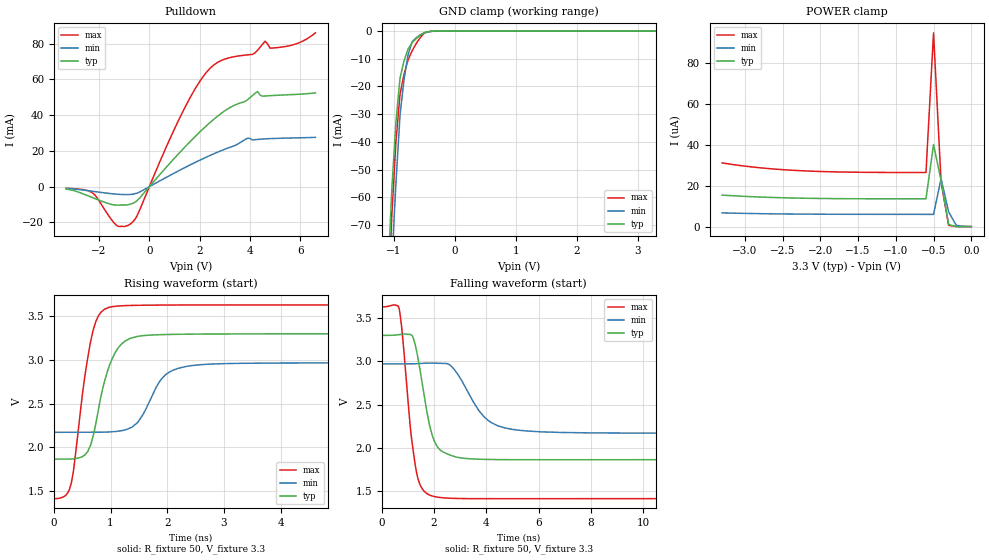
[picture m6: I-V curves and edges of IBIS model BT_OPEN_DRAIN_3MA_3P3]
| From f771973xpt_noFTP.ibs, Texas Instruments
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|   Model Cell BT_OPEN_DRAIN_3MA_3P3
|BT_OPEN_DRAIN_3MA_3P3
[Model]   BT_OPEN_DRAIN_3MA_3P3
Model_type   I/O_open_drain
Polarity   Inverting
Enable   Active-Low
Vinl =  0.8
Vinh =  2
Cref =  15.0000pF
Rref =  100.0000M
Vref =  0V
Vmeas =  1.65
C_comp   3.98845p   2.03906p   4.55356p
[Model Spec]
Vinl   0.8   0.8   0.8
Vinh   2   2   2
[Temperature Range]   25   155   -40
[Voltage Range]   3.3   2.97   3.63
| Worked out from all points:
|   slope of the pulldown table from 0 to 0.495 V, typ, clamps not added: 61.7 ohm
|   GND clamp passes 1 mA (typ) near -0.53 V on its own axis
|   rising waveform, R_fixture 50, V_fixture 3.3: 20-80 % time 326ps typ, 410ps min, 271ps max; typ from 1.87 V to 3.3 V
|   falling waveform, R_fixture 50, V_fixture 3.3: 20-80 % time 525ps typ, 1.02ns min, 426ps max; typ from 3.3 V to 1.86 V
| Nom Voltages:
|   BIASFET=3.3, VDD=1.2, VDDS=3.3, VSS=0
| Min Voltages:
|   BIASFET=2.97, VDD=1.08, VDDS=2.97, VSS=0
| Max Voltages:
|   BIASFET=3.63, VDD=1.32, VDDS=3.63, VSS=0
[POWER_clamp]
|   voltage   I(typ)   I(min)   I(max)
-3.3V     15.41uA    6.707uA    31.17uA
-2.8V     14.47uA    6.332uA    28.78uA
-2.2V     13.87uA    6.102uA    27.25uA
-1.6V     13.64uA    6.016uA    26.64uA
-600mV    13.58uA    5.99uA     26.46uA
-500mV    40.13uA    5.991uA    94.82uA
-400mV    22.54uA    23.52uA    21.76uA
-300mV    969.1nA    7.215uA    616.4nA
-200mV    29.93nA    661.1nA    11.88nA
0V        1.388nA    48.32nA    1.243nA
[Pulldown]
|   voltage   I(typ)   I(min)   I(max)
-3.3V     -1.368mA   -936.2uA   -859.1uA
-2.3V     -5.876mA   -2.477mA   -3.094mA
-1.3V     -10.31mA   -4.18mA    -21.72mA
-800mV    -9.945mA   -4.384mA   -21.31mA
-500mV    -7.961mA   -3.661mA   -16.65mA
1.4V      21.97mA    10.6mA     43.88mA
2.4V      35.71mA    17.39mA    65.97mA
4.3V      53.2mA     26.41mA    76.22mA
4.6V      50.69mA    26.72mA    81.32mA
4.8V      50.87mA    26.86mA    77.39mA
5.4V      51.3mA     27.13mA    78.32mA
6.6V      52.45mA    27.57mA    85.99mA
[GND_clamp]
|   voltage   I(typ)   I(min)   I(max)
-3.3V     -1.746A    -1.481A    -2.454A
-1.1V     -88.72mA   -114.8mA   -101.4mA
-1.033V   -56.66mA   -82.94mA   -65.99mA
-966.7mV  -32.75mA   -54.79mA   -39.79mA
-900mV    -16.98mA   -30.37mA   -22.81mA
-833.3mV  -10.67mA   -17.32mA   -15.58mA
-766.7mV  -6.402mA   -8.477mA   -10.34mA
-700mV    -4.171mA   -3.846mA   -7.085mA
-566.7mV  -1.511mA   -1.331mA   -2.329mA
-500mV    -537.7uA   -639.3uA   -683uA
-300mV    -1.439uA   -12.56uA   -707.1nA
3.3V      1.388nA    14.18uA    1.029nA
[Ramp]
| variable   typ   min   max
dV/dt_f 0.87243134/0.53137713n 0.48603643/1.0377786n   1.344851/0.42962575n
dV/dt_r 0.81373668/0.78906954n 0.45222846/1.5290324n  1.2226949/0.57631885n
R_load = 50
[Rising Waveform]
R_fixture = 50
V_fixture = 3.3
V_fixture_min = 2.97
V_fixture_max = 3.63
|   time   V(typ)   V(min)   V(max)
0s        1.866V     2.173V     1.413V
210.5ps   1.866V     2.173V     1.452V
308.7ps   1.868V     2.173V     1.593V
599.8ps   1.954V     2.173V     3.032V
785.8ps   2.43V      2.173V     3.504V
1.038ns   3.027V     2.179V     3.611V
1.48ns    3.27V      2.287V     3.626V
1.977ns   3.291V     2.834V     3.629V
2.72ns    3.297V     2.952V     3.63V
20.03ns   3.3V       2.97V      3.63V
[Falling Waveform]
R_fixture = 50
V_fixture = 3.3
V_fixture_min = 2.97
V_fixture_max = 3.63
|   time   V(typ)   V(min)   V(max)
0s        3.3V       2.97V      3.63V
667.3ps   3.31V      2.97V      3.606V
1.125ns   3.308V     2.97V      2.146V
1.312ns   3.151V     2.972V     1.745V
1.507ns   2.821V     2.975V     1.546V
1.894ns   2.187V     2.979V     1.446V
2.726ns   1.903V     2.923V     1.415V
3.935ns   1.866V     2.351V     1.411V
4.973ns   1.862V     2.214V     1.411V
20.03ns   1.865V     2.171V     1.413V
